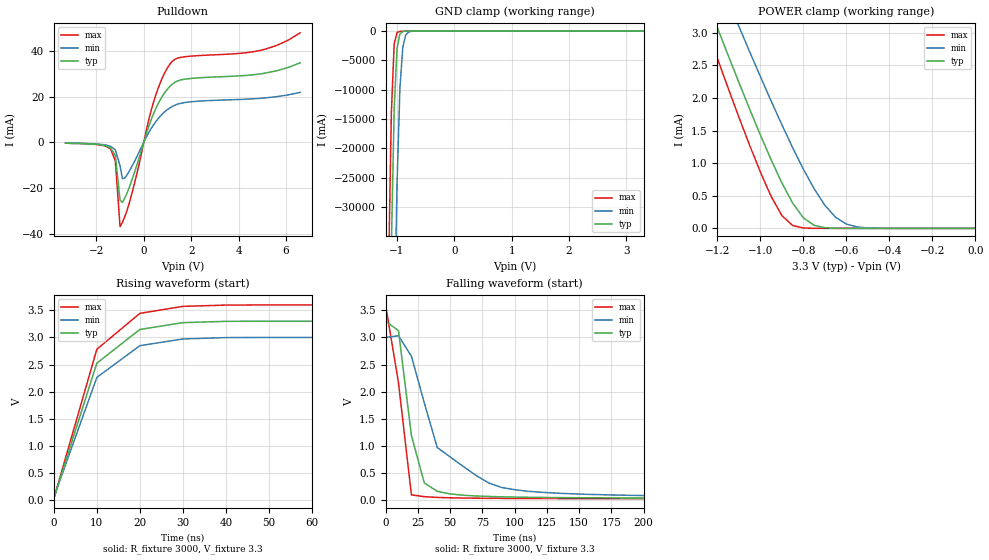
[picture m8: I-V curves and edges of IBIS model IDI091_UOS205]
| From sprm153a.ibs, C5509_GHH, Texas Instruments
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| Pin_model   IDI091_UOS205
[Model]   IDI091_UOS205
 Model_type   I/O_open_drain
 Polarity   Non-Inverting
 Enable   Active-Low
 Vinl  =  1.08
 Vinh  =  2.10
 Vmeas =  1.5
|Variable   typ   min   max
 C_comp   1.868pF   1.855pF   1.87pF
[Temperature Range]   25   125   -40
[Voltage Range]   3.3   3.0   3.6
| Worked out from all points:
|   slope of the pulldown table from 0 to 0.495 V, typ, clamps not added: 34.3 ohm
|   GND clamp passes 1 mA (typ) near -0.59 V on its own axis
|   POWER clamp passes 1 mA (typ) near -0.94 V on its own axis
|   rising waveform, R_fixture 3000, V_fixture 3.3: 20-80 % time 9.31ns typ, 9.83ns min, 8.94ns max; typ from 0.031 V to 3.3 V
|   falling waveform, R_fixture 3000, V_fixture 3.3: 20-80 % time 13.3ns typ, 36.3ns min, 11.9ns max; typ from 3.3 V to 0.031 V
[GND Clamp]
|Voltage   I(typ)   I(min)   I(max)
-3.3V     -2.133kA   -2.174kA   -2.113kA
-1.15V    -70.28A    -122.5A    -42.05A
-1.1V     -36.87A    -85.05A    -14.09A
-1.05V    -13.24A    -51.96A    -2.169A
-1V       -2.863A    -25.89A    -245.7mA
-950mV    -475.9mA   -9.681A    -59.46mA
-900mV    -90.76mA   -2.772A    -35.23mA
-850mV    -29.37mA   -697.5mA   -25.25mA
-800mV    -15.75mA   -174mA     -17.32mA
-600mV    -1.153mA   -2.543mA   -776uA
3.3V      220.7pA    3.118nA    190.5pA
[POWER Clamp]
|Voltage   I(typ)   I(min)   I(max)
-3.3V     21.88mA    21.41mA    22.93mA
-1.25V    3.503mA    4.284mA    3.066mA
-1.2V     3.076mA    3.885mA    2.606mA
-1.1V     2.238mA    3.097mA    1.706mA
-1V       1.432mA    2.327mA    862.5uA
-900mV    697uA      1.589mA    196.2uA
-850mV    388.6uA    1.238mA    44.32uA
-800mV    161.5uA    907.7uA    6.426uA
-700mV    10.42uA    353.6uA    60.52nA
-650mV    1.868uA    169.5uA    5.544nA
-500mV    6.924nA    6.698uA    36.41pA
0V        0A         0A         0A
[Pulldown]
|Voltage   I(typ)   I(min)   I(max)
-3.3V     -300uA     -300uA     -400uA
-1.4V     -2.49mA    -1.77mA    -2.91mA
-1.2V     -5.67mA    -3.29mA    -8.007mA
-1V       -25.36mA   -10.33mA   -36.88mA
-900mV    -26.32mA   -15.83mA   -35.04mA
-800mV    -24.36mA   -15.65mA   -32.55mA
-400mV    -13.45mA   -8.503mA   -18.36mA
450mV     13.4mA     8.177mA    18.82mA
800mV     20.39mA    12.53mA    28.57mA
1.2V      25.39mA    15.67mA    35.37mA
4.9V      29.9mA     19.22mA    40.18mA
6.6V      34.79mA    21.84mA    47.9mA
[Ramp]
|Variable   typ   min   max
 dV/dt_r   2.00V/9.000ns   1.88V/9.000ns   2.16V/9.000ns
 dV/dt_f   2.01V/9.000ns   1.77V/36.000ns   1.98V/5.000ns
 R_load =  3000
[Rising Waveform]
 R_fixture =   3000
 V_fixture =   3.3
 V_fixture_min =  3.0
 V_fixture_max =  3.6
|Time   V(typ)   V(min)   V(max)
0s        30.53mV    46.22mV    23.5mV
10ns      2.526V     2.263V     2.783V
20ns      3.148V     2.849V     3.446V
30ns      3.274V     2.973V     3.575V
40ns      3.298V     2.998V     3.598V
50ns      3.301V     3.001V     3.601V
990ns     3.3V       3V         3.6V
[Falling Waveform]
 R_fixture =   3000
 V_fixture =   3.3
 V_fixture_min =  3.0
 V_fixture_max =  3.6
|Time   V(typ)   V(min)   V(max)
0s        3.3V       3V         3.6V
10ns      3.124V     3.031V     2.162V
20ns      1.192V     2.654V     94.52mV
30ns      314.3mV    1.792V     60.51mV
40ns      160.2mV    969.1mV    46.95mV
80ns      64.84mV    313mV      30.79mV
90ns      58.2mV     229.9mV    29.25mV
110ns     49.64mV    161.1mV    27.3mV
280ns     32.65mV    63.35mV    23.67mV
990ns     30.53mV    46.21mV    23.5mV
